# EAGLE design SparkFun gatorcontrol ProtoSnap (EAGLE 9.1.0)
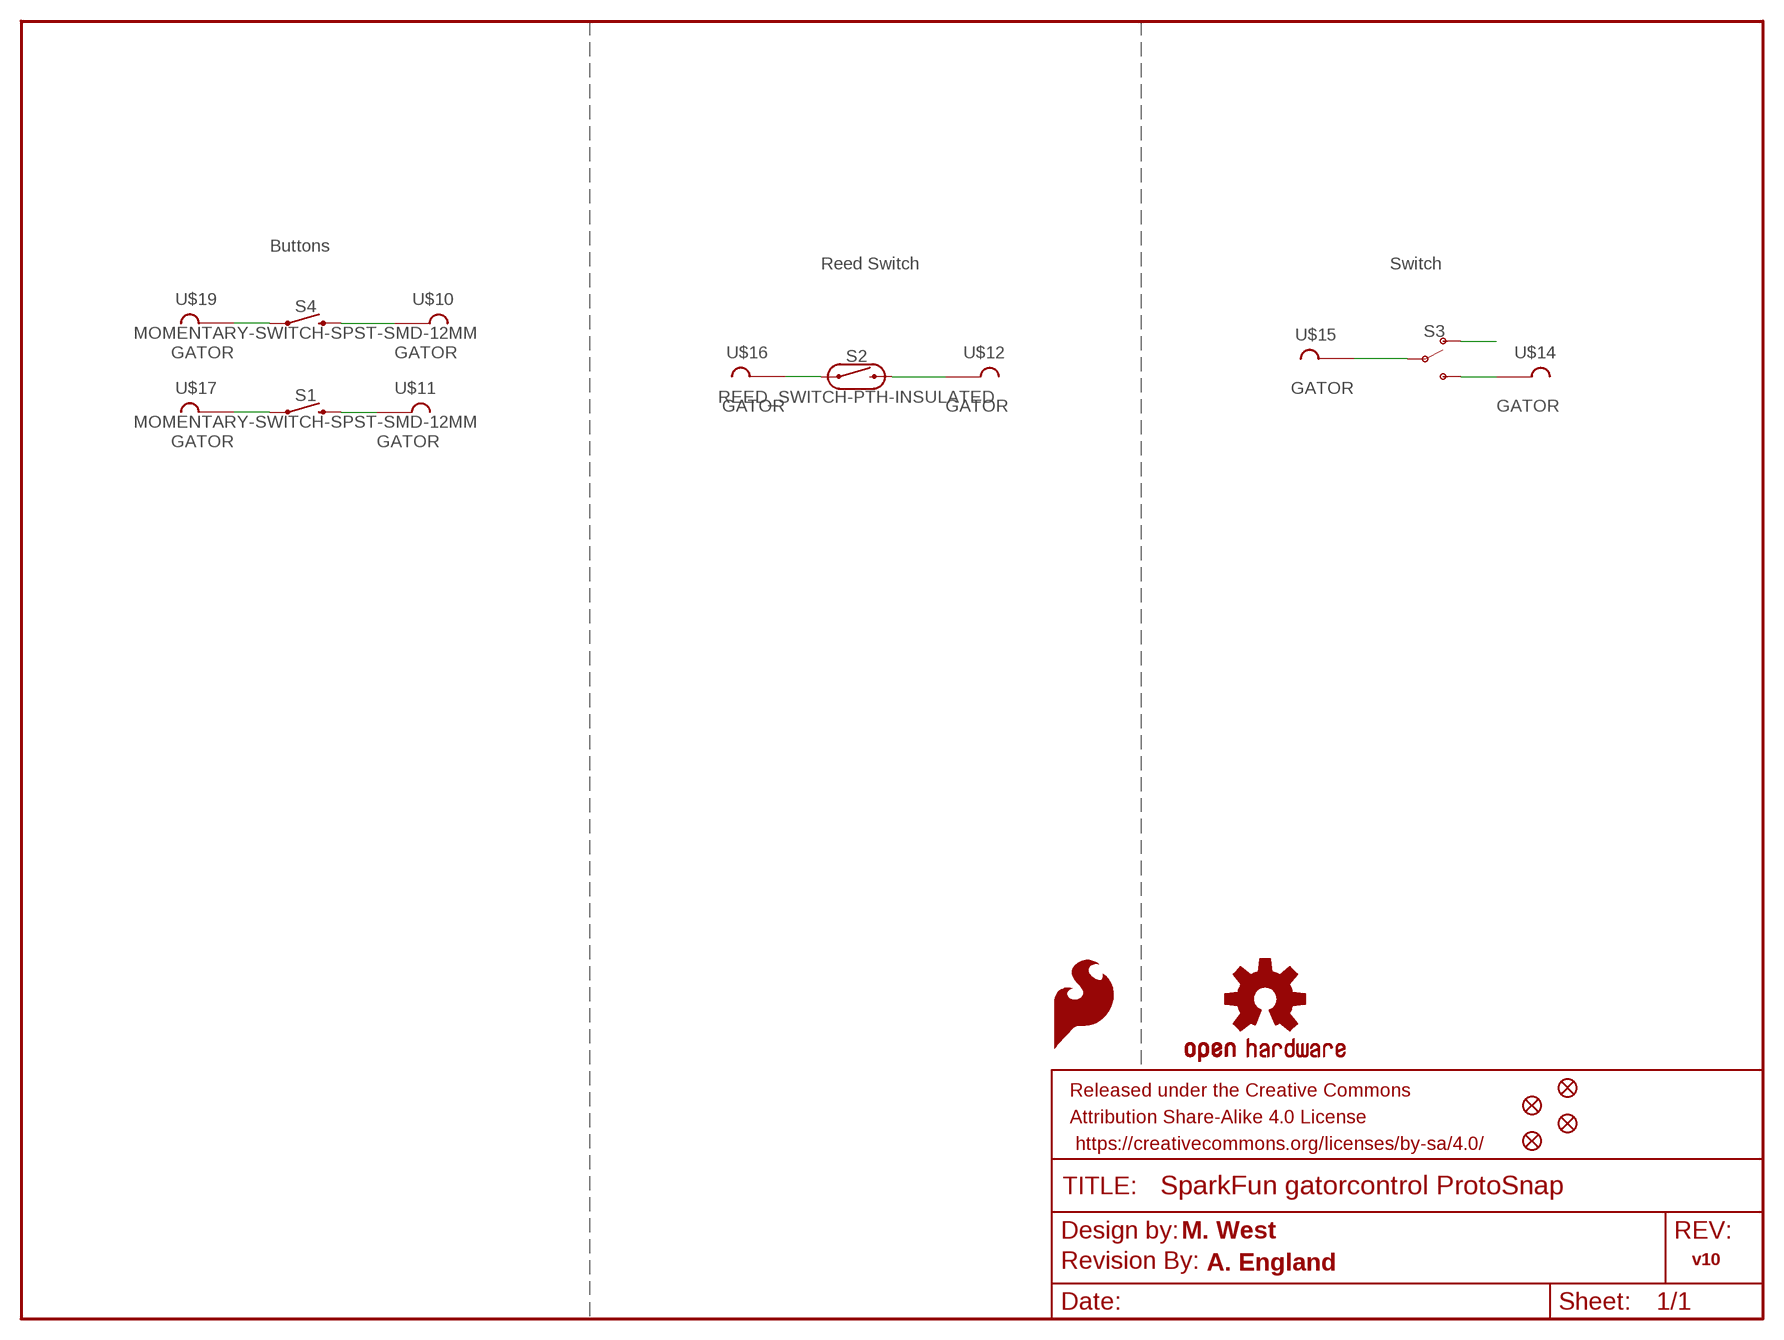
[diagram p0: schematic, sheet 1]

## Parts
FD1  FIDUCIALUFIDUCIAL  [FIDUCIAL-MICRO]
FD2  FIDUCIALUFIDUCIAL  [FIDUCIAL-MICRO]
FD3  FIDUCIALUFIDUCIAL  [FIDUCIAL-MICRO]
FD4  FIDUCIALUFIDUCIAL  [FIDUCIAL-MICRO]
FRAME1  FRAME-LETTER  [CREATIVE_COMMONS]
LOGO1  SFE_LOGO_FLAME.1_INCH  [SFE_LOGO_FLAME_.1]
LOGO2  OSHW-LOGOS  [OSHW-LOGO-S]
LOGO9  REVISION  [REVISION]
S1  MOMENTARY-SWITCH-SPST-SMD-12MM  [TACTILE_SWITCH_SMD_12MM]
S2  REED_SWITCH-PTH-INSULATED  [REED_SWITCH_PLASTIC]
S3  SWITCH-SPDT-SMD-AYZ0202  [SWITCH_DPDT_SMD_AYZ0202]
S4  MOMENTARY-SWITCH-SPST-SMD-12MM  [TACTILE_SWITCH_SMD_12MM]
U$10  GATOR  [GATOR]
U$11  GATOR  [GATOR]
U$12  GATOR  [GATOR]
U$14  GATOR  [GATOR]
U$15  GATOR  [GATOR]
U$16  GATOR  [GATOR]
U$17  GATOR  [GATOR]
U$19  GATOR  [GATOR]

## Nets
N$1: S4.1 U$19.P$1 U$19.P$2
N$2: S4.3 U$10.P$1 U$10.P$2
N$3: S1.1 U$17.P$1 U$17.P$2
N$4: S1.3 U$11.P$1 U$11.P$2
N$5: S2.P$1 U$16.P$1 U$16.P$2
N$6: S2.P$2 U$12.P$1 U$12.P$2
N$7: S3.2(P) U$15.P$1 U$15.P$2
N$8: S3.1(O)
N$9: S3.3(S) U$14.P$1 U$14.P$2

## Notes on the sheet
- Buttons
- Reed Switch | Switch
- M. West
- v10
- A. England

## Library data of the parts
FD1-FD4 = SparkFun-Aesthetics:FIDUCIAL: Fiducial Alignment Points
FRAME1 = SparkFun-Aesthetics:FRAME-LETTER: Schematic Frame - Letter
LOGO1 = SparkFun-Aesthetics:SFE_LOGO_FLAME: SparkFun Flame Logo
LOGO2 = SparkFun-Aesthetics:OSHW-LOGO: Open-Source Hardware (OSHW) Logo
LOGO9 = SparkFun-Aesthetics:REVISION: "Revision By" Text
S1 S4 = SparkFun-Switches:MOMENTARY-SWITCH-SPST: Momentary Switch (Pushbutton) - SPST; PROD_ID: SWCH-11967; SF_SKU: COM-12993
S2 = SparkFun-Switches:REED_SWITCH: Reed Switch; PROD_ID: SWCH-10467; SF_SKU: COM-10601
S3 = SparkFun-Switches:SWITCH-SPDT: Single Pole, Double Throw (SPDT) Switch Single-pole, double-throw (SPDT) switch. Variant Overview SMD-AYZ0202 Surface Mount DPDT Switch (COM-00597) Used on e.g. LilyPad Arduino USB - ATmega32U4 Board PTH-11.6X4.0MM SPDT Mini Power Switch (COM-00102) Used on e.g. SparkFun Simon Says - Through-Hole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; PROD_ID: SWCH-08179; SF_ID: COM-00597
U$10-U$12 U$14-U$17 U$19 = SparkFun-Connectors:GATOR

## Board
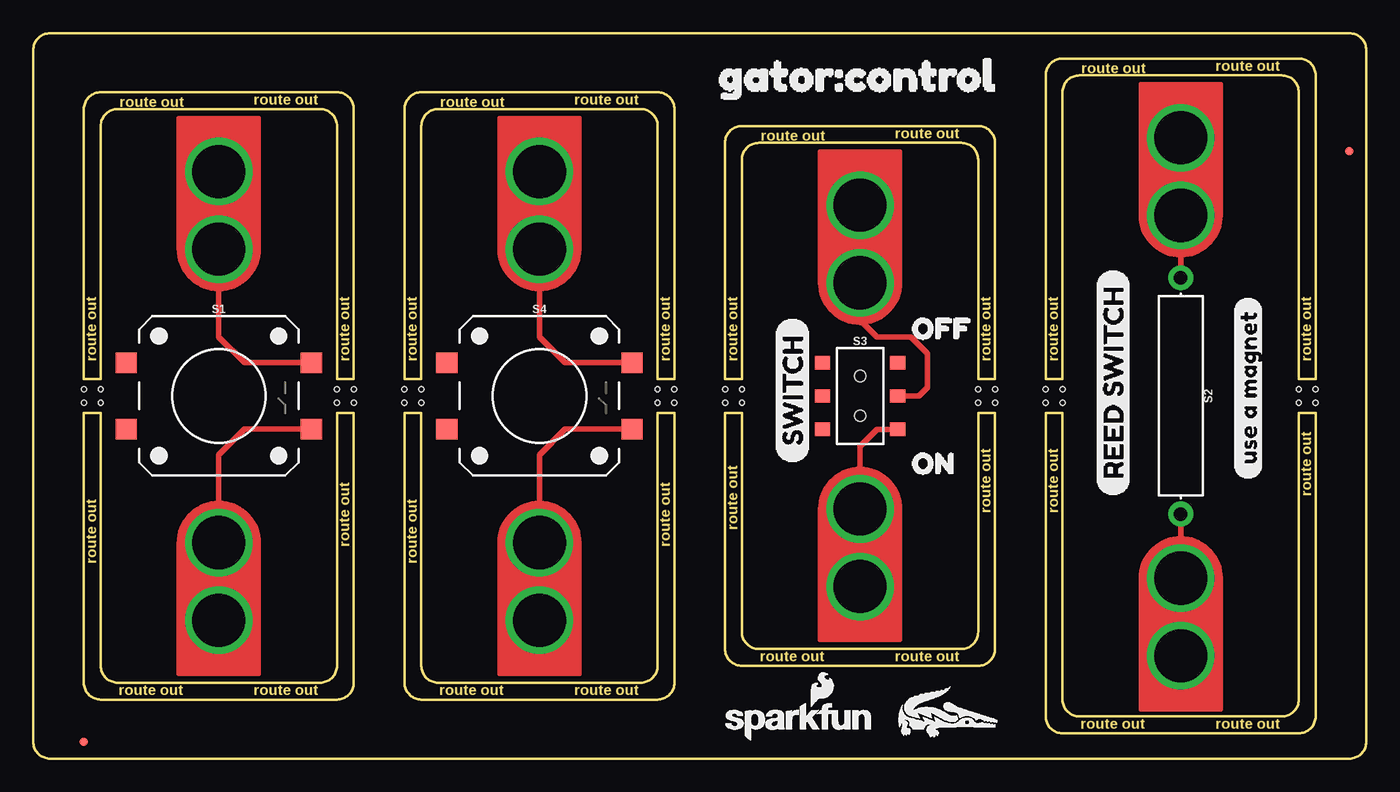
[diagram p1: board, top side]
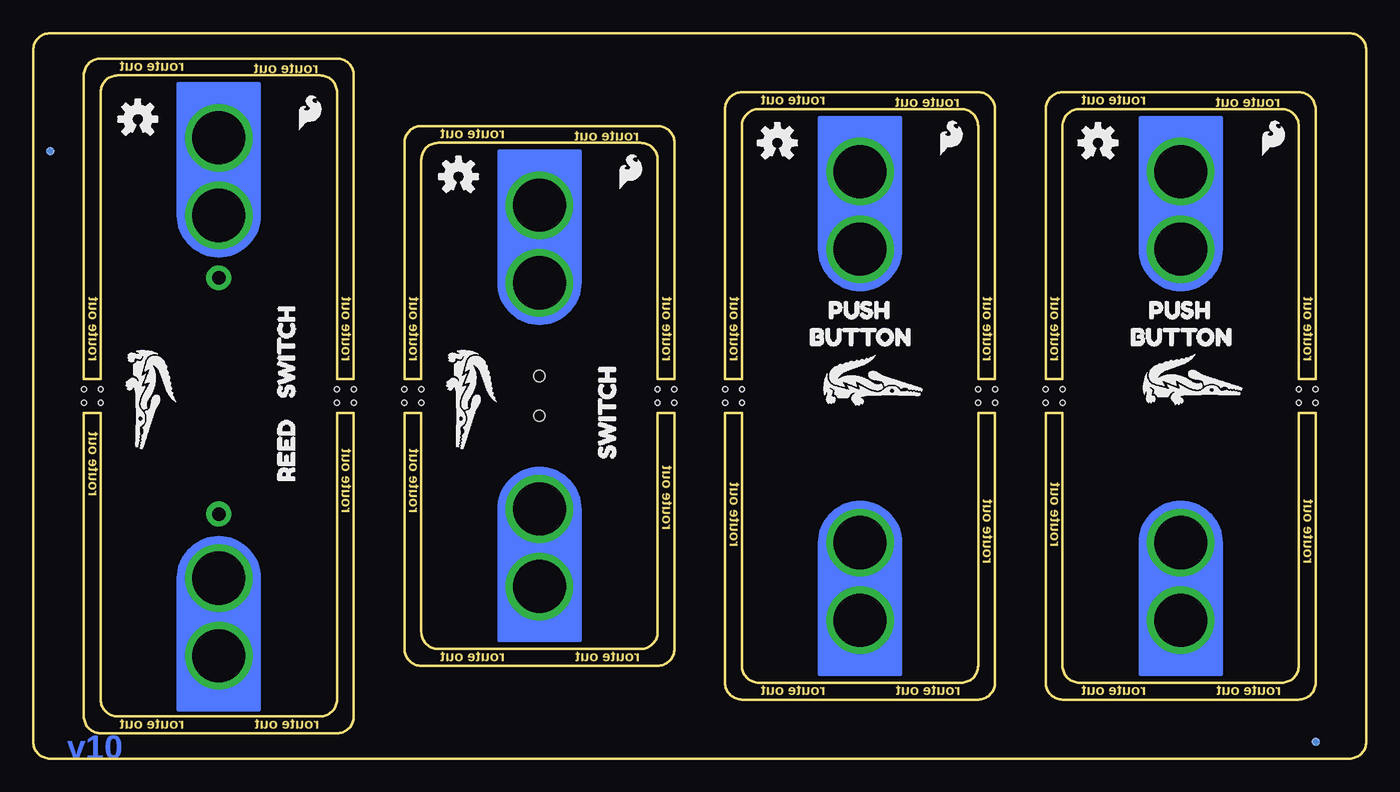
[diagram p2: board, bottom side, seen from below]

Size 100.33 x 54.61 mm. Coordinates in mm from the lower left corner, seen from the top.
Outline: 120 segments
Copper layers (1*16): Top 0.035mm / dielectric 1.5mm / Bottom 0.035mm
Design rules "SparkFun-2-layer-TIGHT": minimum track width 7mil, minimum drill 15mil, track to track 7mil, track to pad 7mil, pad to pad 7mil, via to via 7mil, smd to smd 7mil, copper to edge 7mil, drill to drill 7mil, minimum pad ring 7mil, minimum via ring 7mil, stop-mask expansion 4mil, vias tented up to drill 25mil, thermal gap 10mil
Holes 0.38 mm at 95.25,27.81 95.25,26.8 77.47,26.8 77.47,27.81 53.34,26.8 53.34,27.81 46.99,26.8 46.99,27.81 29.21,26.8 29.21,27.81 22.86,26.8 22.86,27.81 5.08,26.8 5.08,27.81 27.94,27.81 27.94,26.8 24.13,27.81 24.13,26.8 3.81,27.81 3.81,26.8 48.26,27.81 48.26,26.8 52.07,27.81 52.07,26.8 76.2,27.81 72.39,27.81 71.12,27.81 76.2,26.8 72.39,26.8 71.12,26.8 96.52,27.81 96.52,26.8

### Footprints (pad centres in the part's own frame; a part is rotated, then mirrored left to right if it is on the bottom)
FIDUCIAL-MICRO = smd 0.635 x 0.635: 1 0,0
TACTILE_SWITCH_SMD_12MM = smd 1.6 x 1.55: 1 6.975,-2.5; 2 -6.975,-2.5; 3 6.975,2.5; 4 -6.975,2.5
REED_SWITCH_PLASTIC = drill 1.016 pad 1.88: P$1 -8.89,0; P$2 8.89,0
SWITCH_DPDT_SMD_AYZ0202 = smd 1 x 1.15: 1 -2.5,2.825; 2 0,2.825; 3 2.5,2.825; 4 -2.5,-2.825; 5 0,-2.825; 6 2.5,-2.825 | hole 0.85: 1.5,0; -1.5,0
GATOR = drill 4 pad 5.08: P$1 0,-6.096; P$2 0,-0.254

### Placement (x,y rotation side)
FD1  99.06,45.72 0 top
FD2  99.06,45.72 0 bottom
FD3  3.81,1.27 0 bottom
FD4  3.81,1.27 0 top
FRAME1  not placed on the board
LOGO1  56.52,42.55 0 bottom
LOGO2  68.33,43.81 0 bottom
LOGO3  OSHW-LOGOS  [OSHW-LOGO-S]  44.32,46.35 0 bottom
LOGO4  SFE_LOGO_FLAME.1_INCH  [SFE_LOGO_FLAME_.1]  32.38,45.09 0 bottom
LOGO5  OSHW-LOGOS  [OSHW-LOGO-S]  20.19,46.35 0 bottom
LOGO6  SFE_LOGO_FLAME.1_INCH  [SFE_LOGO_FLAME_.1]  8.13,45.09 0 bottom
LOGO7  SFE_LOGO_FLAME.1_INCH  [SFE_LOGO_FLAME_.1]  80.64,46.99 0 bottom
LOGO8  OSHW-LOGOS  [OSHW-LOGO-S]  92.46,48.13 0 bottom
LOGO9  not placed on the board
S1  13.97,27.3 0 top
S2  86.36,27.3 270 top
S3  62.23,27.3 270 top
S4  38.1,27.3 0 top
U$1  [GATOR#PNG]  91.38,27.37 270 bottom
U$2  [BUTTON3]  18.92,31.75 0 bottom
U$3  [PUSH4]  17.53,33.78 0 bottom
U$4  [PUSH4]  41.66,33.78 0 bottom
U$5  [BUTTON3]  43.05,31.75 0 bottom
U$6  [OFF9]  64.77,32.38 0 top
U$7  [REED_SWITCH0]  81.28,19.68 90 top
U$8  [SWITCH2]  57.15,22.23 90 top
U$9  [USE_A_MAGNET10]  91.44,20.95 90 top
U$10  38.1,38.1 180 top
U$11  13.97,38.1 180 top
U$12  86.36,13.84 0 top
U$13  [ON8]  64.77,22.23 0 top
U$14  62.23,19.05 0 top
U$15  62.23,35.56 180 top
U$16  86.36,40.64 180 top
U$17  13.97,16.51 0 top
U$18  [SWITCH5]  57.15,21.46 90 bottom
U$19  38.1,16.51 0 top
U$20  [REED6]  81.28,19.68 90 bottom
U$21  [SWITCH5]  81.28,26.04 90 bottom
U$22  [GATOR#PNG]  68.52,3.62 0 top
U$23  [GATOR#CONTROL0]  49.53,51.44 0 top
U$24  [SFE_LOGO_NAME_FLAME_.1]  51.69,1.27 0 top
U$28  [GATOR#PNG]  37.47,28.57 0 bottom
U$29  [GATOR#PNG]  67.25,27.37 270 bottom
U$33  [ORDERING_INSTRUCTIONS]  not placed on the board
U$70  [GATOR#PNG]  13.4,28.64 0 bottom

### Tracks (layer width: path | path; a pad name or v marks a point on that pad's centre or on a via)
N$1
  Top 0.203: U$19.P$2 U$19.P$1
  Top 0.406: U$19.P$2 38.1,22.86 40.05,24.8 S4.1
N$2
  Top 0.203: U$10.P$1 38.1,38.1 U$10.P$2
  Top 0.406: U$10.P$1 38.1,42.77 | S4.3 40.05,29.8 38.1,31.75 38.1,38.1
N$3
  Top 0.203: U$17.P$2 U$17.P$1
  Top 0.406: S1.1 15.91,24.8 13.97,22.86 U$17.P$2
N$4
  Top 0.203: U$11.P$1 13.97,38.1 U$11.P$2
  Top 0.406: S1.3 15.91,29.8 13.97,31.75 13.97,38.1
N$5
  Top 0.203: U$16.P$2 86.36,40.64
  Top 0.406: 86.36,39.37 86.36,40.64 | 86.36,40.64 U$16.P$1 | S2.P$1 86.36,40.64
N$6
  Top 0.406: S2.P$2 86.36,15.24 | 86.36,15.24 U$12.P$1 | U$12.P$2 86.36,15.24
N$7
  Top 0.203: 62.23,33.02 U$15.P$1 62.23,38.99 61.98,38.73
  Top 0.406: 60.96,38.73 61.98,38.73 62.1,38.73 62.11,38.73 | S3.2 66.67,27.3 67.31,27.94 67.31,30.48 66.04,31.75 63.5,31.75 62.23,33.02 U$15.P$2
N$9
  Top 0.406: S3.3 65.02,24.77 63.5,24.77 62.23,23.5 62.23,17.78 U$14.P$2 U$14.P$1

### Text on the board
Bottom: v10
Dimension: route out | route out | route out | route out | route out | route out | route out | route out | route out | route out | route out | route out | route out | route out | route out | route out | route out | route out | route out | route out | route out | route out | route out | route out | route out | route out | route out | route out | route out | route out | route out | route out
tDocu: M. West | A. England | Solder Mask: Black Gloss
